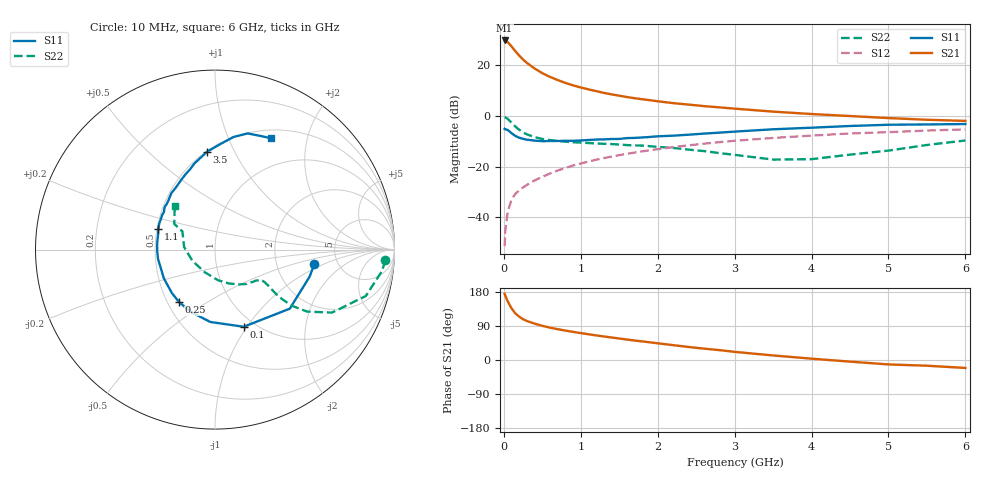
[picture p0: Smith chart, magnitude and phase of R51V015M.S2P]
! SIEMENS Small Signal Semiconductors
! BFR183
! Si NPN RF Bipolar Junction Transistor in SOT23
! VCE = 1 V  IC = 15 mA
! Common Emitter S-Parameters:  May  1996
# GHz  S  MA  R  50
!  f  S11  S21  S12  S22
! GHz  MAG  ANG  MAG  ANG  MAG  ANG  MAG  ANG
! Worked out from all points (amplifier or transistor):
!   36 points, 10 MHz to 6 GHz, reference 50 ohm
!   highest |S21| = 29.8 dB at 10 MHz (marker M1)
!   |S21| within 3 dB of that: start of sweep to 117 MHz
!   unconditionally stable (mu >= 1): 503.2 MHz to 2.693 GHz
!   at 250 MHz: K = 0.77, MSG = 25.2 dB, |S12| = -28.2 dB
!   at 1.4 GHz: K = 1.07, MAG = 10.6 dB, |S12| = -16.0 dB
!   at 6 GHz: K = 0.94, MSG = 1.7 dB, |S12| = -5.3 dB
!   S11 on the Smith chart (normalised r, x): 10 MHz: 3.33, -0.79; 100 MHz: 0.89, -0.97; 250 MHz: 0.57, -0.39; 1.1 GHz: 0.51, +0.13; 3.5 GHz: 0.50, +0.79; 6 GHz: 0.61, +1.45
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0.01  0.5591 -8.4  31 174.7  0.0027 87.8  0.951 -3.6
0.02  0.5482 -16.0  30.88 169.3  0.0056 83.9  0.9381 -7.3
0.05  0.531 -38.3  28.8 154.9  0.0128 75.2  0.8792 -17.1
0.1  0.4587 -69.6  23.65 136.3  0.0225 66.1  0.7404 -28.3
0.15  0.404 -93.7  18.99 122.8  0.0291 63.5  0.6194 -33.9
0.2  0.3732 -110.5  15.61 114.2  0.0341 62.5  0.5356 -36.0
0.25  0.3548 -124.1  13.01 107.7  0.039 62.3  0.4766 -36.4
0.3  0.3412 -134.7  11.17 102.8  0.0437 63.7  0.4346 -36.3
0.4  0.3269 -150.6  8.673 96.0  0.0535 64.9  0.383 -35.0
0.5  0.3189 -162.1  7.012 90.2  0.063 66.2  0.3532 -33.9
0.6  0.3215 -170.4  5.921 85.4  0.0734 66.7  0.3347 -33.4
0.7  0.3222 -178.3  5.125 81.3  0.084 67.0  0.3221 -33.2
0.8  0.3236 175.5  4.501 77.6  0.0944 66.8  0.3116 -33.4
0.9  0.3249 170.3  4.025 74.2  0.1055 66.7  0.3038 -33.6
1.1  0.3362 160.3  3.356 68.0  0.1265 65.6  0.2933 -35.9
1.3  0.3457 150.9  2.864 62.1  0.1477 64.0  0.2829 -38.0
1.6  0.3667 140.1  2.367 53.9  0.1797 61.2  0.2669 -43.2
2.2  0.4093 122.0  1.797 39.2  0.2431 54.5  0.2343 -56.2
3.5  0.5473 94.6  1.221 12.0  0.369 37.0  0.1381 -115.1
4.5  0.6358 80.7  0.999 -4.3  0.4524 23.7  0.1729 175.1
5.5  0.6821 68.2  0.844 -15.1  0.5163 11.7  0.2683 147.8
6  0.6948 63.1  0.801 -21.0  0.545 4.2  0.3292 133.0
